(* Logix 5000 Routine export SpecLink_Routine; software revision 36.00 *)

TYPE DUT_NDSN_spLink :   // UDDT that holds the Cyclic and ACyclic data for the SpectraLink.
STRUCT
   b_r_LostComm : BOOL;
   b_r_PLC_CommReadOnly : BOOL;
   b_r_SystemReady : BOOL;   // Pattern Status Word 0 Bit 0
   b_r_Fault : BOOL;   // Pattern Status Word 0 Bit 1
   b_r_Alert : BOOL;   // Pattern Status Word 0 Bit 2
   b_r_Commissioned : BOOL;   // Pattern Status Word 0 Bit 3
   b_r_RecipeModified : BOOL;   // Pattern Status Word 0 Bit 5
   i_r_Recipe : INT;
   i_r_PalletizedCount : INT;
   i_r_PalletizedSkipCount : INT;
   di_r_App_Trig_ProductCount : DINT;
   di_r_FeedCount : DINT;
   di_r_DeliveryCount : DINT;
   st_r_AppStat : DUT_NDSN_spLink_Chan_Status[8];
   st_r_TrigStat : DUT_NDSN_spLink_Trig_Status[8];
   st_r_EncoStat : DUT_NDSN_spLink_Encoder_Status[8];
   i_r_ProductLength : DINT[8];
   i_r_ProdRate : INT;
   i_r_LineSpeed : INT[2];   // m/min units
   i_r_RunupOutput : INT[2];
   b_w_UnitEnable : BOOL;   // Pattern Control Word 0 Bit 0
   b_w_ClearAllAlarms : BOOL;   // Clear all System Faults and Alerts (Rising Edge).
   b_w_ResetAllCounters : BOOL;   // Reset all counters (rising edge).
   i_w_LoadRecipe : INT;
   i_w_PalletizedCount : INT;   // Write 0 to decrement; 1 to increment; 2 to reset; else does nothing.
   i_w_PalletizedSkipCount : INT;   // Write 0 to decrement; 1 to increment; 2 to reset; else does nothing.
   di_w_App_Trig_ProductCount : DINT;
   di_w_FeedCountReset : DINT;
   di_w_DeliveryCountReset : DINT;
   st_w_AppCtl : DUT_NDSN_spLink_Chan_CTL[8];
   st_rw_BeadAgg : DUT_NDSN_spLink_Bead[8];
   i_rw_RnUpPercentOutP1 : INT[2];
   i_rw_RnUpLineSpdP1 : INT[2];
   i_rw_RnUpPercentOutP2 : INT[2];
   i_rw_RnUpLineSpdP2 : INT[2];
   i_rw_RnUpLowLim : INT[2];
   i_rw_RnUpHighLim : INT[2];
   di_rw_EncoderRes : DINT[2];
   i_rw_TriggerMaskDist : DINT[8];
   i_rw_TriggerChCtl : INT[8];
   i_rw_EncoderChCtl : INT[2];
   i_rw_RandAdjStart : INT[8];
   i_rw_RandAdjEnd : INT[8];
   i_rw_VirtualTriggerSize : DINT[8];
   i_rw_ContStartSpeed : INT[8];
   i_rw_ContStopSpeed : INT[8];
   i_rw_ContKnifeCutDelay : DINT[8];
   i_rw_ContKnifeCutGap : DINT[8];
   di_rw_GTO : DINT[8];
   i_r_ErrorInfo : INT[4];
   i_r_SpecCtl : INT[4];
   i_r_CurrentFault : INT;
END_STRUCT
END_TYPE

TYPE DUT_NDSN_spLink_Bead :
STRUCT
   di_rw_NumOfBeads : DINT;
   di_rw_BeadDelay : DINT[8];   // 1/4 mm
   di_rw_BeadDuration : DINT[8];   // 1/4 mm
   di_rw_mode : DINT;   // 1/4 mm
   di_rw_MaxGunTime : DINT;   // microseconds
   di_rw_LineSpeedActivation : DINT;   // 100th m/min
   di_rw_LineSpeedDeactivation : DINT;   // 100th m/min
   di_rw_Interval : DINT;   // 1/4 mm
   di_rw_AdhesiveSavings : DINT;   // 30%-60%
   di_rw_EcoBeadPattern : DINT;   // 0-40, Illegal values: 0,1,11,20,21,30,31,38,39
END_STRUCT
END_TYPE

TYPE DUT_NDSN_spLink_Chan_CTL :
STRUCT
   b_w_Enable : BOOL;
   b_w_Purge : BOOL;
END_STRUCT
END_TYPE

TYPE DUT_NDSN_spLink_Chan_Status :
STRUCT
   b_r_Enabled : BOOL;
   b_r_Fault : BOOL;
   b_r_Alert : BOOL;
   b_r_Output_Active : BOOL;
   b_r_Installed : BOOL;
END_STRUCT
END_TYPE

TYPE DUT_NDSN_spLink_Encoder_Status :   // SpectraLink Encoder Channel Status
STRUCT
   b_r_Missing : BOOL;
   b_r_Phase_Missing : BOOL;
   b_r_Scaled : BOOL;
   b_r_Fault : BOOL;
   b_r_Alert : BOOL;
   b_r_Installed : BOOL;
END_STRUCT
END_TYPE

TYPE DUT_NDSN_spLink_HMI_Data :
STRUCT
   r_w_RunUp_1_P1_LineSpeed : REAL;
   r_w_RunUp_2_P1_LineSpeed : REAL;
   r_w_RunUp_1_P2_LineSpeed : REAL;
   r_w_RunUp_2_P2_LineSpeed : REAL;
   r_tempstorage : REAL[4];
   i_tempstorage : INT[4];
END_STRUCT
END_TYPE

TYPE DUT_NDSN_spLink_Rd_Wt :
STRUCT
   i_arr_ReadValue : INT[60];
   i_ReadADI : INT;
   b_ReadDone : BOOL;
   i_arr_WriteValue : INT[60];
   i_WriteADI : INT;
   i_WriteSizeBytes : INT;
   b_WriteEvent : BOOL;
   b_WriteDone : BOOL;
   b_FirstScan : BOOL;
   b_AllowWrites : BOOL;
   b_WriteErr : BOOL;
   b_ReadErr : BOOL;
END_STRUCT
END_TYPE

TYPE DUT_NDSN_spLink_Trig_Status :   // SpectraLink Trigger Channel Status
STRUCT
   b_r_Detected : BOOL;
   b_r_Fault : BOOL;
   b_r_Alert : BOOL;
   b_r_Active : BOOL;
   b_r_Installed : BOOL;
END_STRUCT
END_TYPE

TYPE DUT_spLink_ADI :
STRUCT
   i_ADI : INT;
   i_Size : INT;
END_STRUCT
END_TYPE

ADD_ON_INSTRUCTION AOI_spLink   (* revision 1.0 *)
// AOI to handle the I/O based data (Default Data) and Acyclic Data (low Priority) from the SpectraLink Pattern Controller.
VAR_IN_OUT
   IO_Input : INT[64]; {required}
   IO_Out : INT[64]; {required}
   spLink_HMI : DUT_NDSN_spLink; {required}
   IO_AcycRdWt : DUT_NDSN_spLink_Rd_Wt; {required}
   ReadMsg : MESSAGE; {required}
   WriteMsg : MESSAGE; {required}
   Read_Buffer : INT[100]; {required}
   Write_Buffer : INT[100]; {required}
END_VAR
VAR
   st_ADI_List : DUT_spLink_ADI[40]; {access None}
   tm_Command : FBD_TIMER; {access None}
   tm_Acyc : FBD_TIMER; {access None}
   b_AdhesiveOn : BOOL; {access None}
   b_AdhesiveOff : BOOL; {access None}
   b_Read : BOOL; {access None}
   i_ADI_Range : INT; {access None}
   i_ADI_Size : INT := 20; {access None}
   i_CompareIndex : INT; {access None}
   i_Index : INT; {access None}
   i_Index_Write : INT; {access None}
   i_rwADI_Count : INT := 12; {access None}
   i_rwDataSize : INT := 24; {access None}
   i_Size : INT; {access None}
   i_SizeofStruct : INT := 48; {access None}
   i_ValueIndex : INT; {access None}
   i : INT; {access None}
   i_temp_CPC : INT; {access None}
   arr_WriteIndex : DINT[40]; {access None}
   arr_WriteStartingAddress : DINT[40]; {access None}
   b_AcycWT_Rising : BOOL; {access None}
   arr_HMI : INT[600]; {access None}
   arr_HMI_Buffer : INT[600]; {access None}
   arr_HMI_Compare : INT[600]; {access None}
   b_AcycRD_Rising : BOOL; {access None}
   b_CommandRising : BOOL; {access None}
   tm_PalletizedCount_Reset : FBD_TIMER; {access None}
   b_ResetCurrentPalletizedCount : BOOL; {access None}
   b_ResetCurrentPalletizedSkipCount : BOOL; {access None}
   tm_PalletizedSkipCount_Reset : FBD_TIMER; {access None}
   i_temp_CPSC : INT; {access None}
   i_LoopCnt : INT; {access None}
   b_ResetSelectCount : BOOL; {access None}
   tm_ResetSelectCount : FBD_TIMER := (PRE := 5000); {access None}
   TRUE : BOOL := 1; {access None}
   FALSE : BOOL; {access None}
   tm_ResetFeedCount : FBD_TIMER; {access None}
   tm_ResetDeliveryCount : FBD_TIMER; {access None}
   i_WriteSizeTemp : INT; {access None}
   i_ReadADI_Temp : INT; {access None}
   tm_WriteEvent : FBD_TIMER; {access None}
   b_WriteEventONS : BOOL; {access None}
   i_WritePtr : DINT; {access None}
   Read_Watchdog : FBD_TIMER; {access None}
   Read_Time_Tic : FBD_TIMER; {access None}
   DINT_TEMP : DINT; {access None}
   DINT_Offset : INT; {access Read Only}
END_VAR

ROUTINE Logic   (* structured text *)
   //
   //		SpectraLink Add-On Instruction used to read/write Cyclic (high priority I/O)
   //		and Acyclic (low priority) data.
   //
   //
   //*******************************************************************************
   //	Initialize Code
   //*******************************************************************************
   
   IF IO_AcycRdWt.b_FirstScan THEN
   	i_ADI_Size:= 29;
   	i_rwADI_Count :=26;
   	i_SizeofStruct := 531;
   	i_rwDataSize := 522;
   	i_ADI_Range := 0;
   	i_ValueIndex :=0;
   	i_Index:=0;
   	IO_AcycRdWt.b_FirstScan := 0;		//Reset the FirstScan bit sent to the ADI from the main routine.
   	IO_AcycRdWt.b_AllowWrites := 0;		//Cycle through the full Read Data Set before allowing Writes to occur.  This populates the write compare buffers.
   
   	FOR i := 0 TO i_rwADI_Count DO
   		i_ADI_Range := i_ADI_Range + st_ADI_List[i].i_Size;
   		arr_WriteIndex[i] := i_ADI_Range;					//Index of all Read/Write ADI
   		arr_WriteStartingAddress[i + 1] := i_ADI_Range;		//All Read/Write ADI Starting Address
   	END_FOR;
   
   
   END_IF;
   
   
   
   
   //*******************************************************************************
   //  Start of Cyclic Data Code
   //
   //	The following code handles the I/O data for the High Priority DEFAULT ADIs.
   //*******************************************************************************
   
   // SpectraLink system Status
   spLink_HMI.b_r_SystemReady := IO_Input[0].0;
   spLink_HMI.b_r_Fault := IO_Input[0].1;
   spLink_HMI.b_r_Alert := IO_Input[0].2;
   spLink_HMI.b_r_Commissioned := IO_Input[0].3;
   spLink_HMI.b_r_PLC_CommReadOnly := IO_Input[0].4;
   spLink_HMI.b_r_RecipeModified := IO_Input[0].5;
   
   spLink_HMI.i_r_Recipe := IO_Input[4];
   spLink_HMI.i_r_PalletizedCount := IO_Input[5];
   spLink_HMI.i_r_PalletizedSkipCount := IO_Input[6];
   
   COP(IO_Input[7], spLink_HMI.di_r_App_Trig_ProductCount, 6);
   
   // Copy the Applicator Status Structure Bits from the IO_Inputs
   i_LoopCnt := 0;
   While (i_LoopCnt < 8) DO
   	spLink_HMI.st_r_AppStat[i_LoopCnt].b_r_Enabled := IO_Input[13+i_LoopCnt].0;
   	spLink_HMI.st_r_AppStat[i_LoopCnt].b_r_Fault := IO_Input[13+i_LoopCnt].1;
   	spLink_HMI.st_r_AppStat[i_LoopCnt].b_r_Alert := IO_Input[13+i_LoopCnt].2;
   	spLink_HMI.st_r_AppStat[i_LoopCnt].b_r_Output_Active := IO_Input[13+i_LoopCnt].3;
   	spLink_HMI.st_r_AppStat[i_LoopCnt].b_r_Installed := IO_Input[13+i_LoopCnt].4;
   	i_LoopCnt := i_LoopCnt+1;
   end_while;
   
   // Copy the Trigger Status Structure Bits from the IO_Inputs
   i_LoopCnt := 0;
   While (i_LoopCnt < 8) DO
   	spLink_HMI.st_r_TrigStat[i_LoopCnt].b_r_Detected := IO_Input[21+i_LoopCnt].0;
   	spLink_HMI.st_r_TrigStat[i_LoopCnt].b_r_Fault := IO_Input[21+i_LoopCnt].1;
   	spLink_HMI.st_r_TrigStat[i_LoopCnt].b_r_Alert := IO_Input[21+i_LoopCnt].2;
   	spLink_HMI.st_r_TrigStat[i_LoopCnt].b_r_Active := IO_Input[21+i_LoopCnt].3;
   	i_LoopCnt := i_LoopCnt+1;
   end_while;
   
   // Copy the Encoder Status Structure Bits from the IO_Inputs
   i_LoopCnt := 0;
   While (i_LoopCnt < 2) DO
   	spLink_HMI.st_r_EncoStat[i_LoopCnt].b_r_Missing := IO_Input[29+i_LoopCnt].0;
   	spLink_HMI.st_r_EncoStat[i_LoopCnt].b_r_Phase_Missing := IO_Input[29+i_LoopCnt].1;
   	spLink_HMI.st_r_EncoStat[i_LoopCnt].b_r_Scaled := IO_Input[29+i_LoopCnt].2;
   	spLink_HMI.st_r_EncoStat[i_LoopCnt].b_r_Fault := IO_Input[29+i_LoopCnt].3;
   	spLink_HMI.st_r_EncoStat[i_LoopCnt].b_r_Alert := IO_Input[29+i_LoopCnt].4;
   	i_LoopCnt := i_LoopCnt+1;
   end_while;
   
   
   //******************************************************************************************************************
   //Adjust the Product Length by a factor of 4
   //******************************************************************************************************************
   
   i_LoopCnt := 0;
   While (i_LoopCnt < 8) DO
   	DINT_Offset := i_LoopCnt*2;
   	COP(IO_Input[31+DINT_Offset], DINT_TEMP, 2);
   	spLink_HMI.i_r_ProductLength[i_LoopCnt] := (DINT_TEMP/4);
   	i_LoopCnt := i_LoopCnt+1;
   end_while;
   
   
   COP(IO_Input[47], spLink_HMI.i_r_ProdRate, 1);
   COP(IO_Input[48], spLink_HMI.i_r_LineSpeed[0], 2);
   COP(IO_Input[50], spLink_HMI.i_r_RunupOutput[0], 2);
   
   
   //******************************************************************************************************************
   //Cyclic WRITE Section
   //******************************************************************************************************************
   
   IO_Out[0].0 := spLink_HMI.b_w_UnitEnable;
   IO_Out[2].0 := spLink_HMI.b_w_ClearAllAlarms;
   IO_Out[2].1 := spLink_HMI.b_w_ResetAllCounters;
   
   IO_Out[4] := spLink_HMI.i_w_LoadRecipe;
   
   
   //********************************************************************************************************************************
   //Current Palatized Count & Current Palatized Skip Count     increment (1) or decrement (0);  else = other value     (ADI 16359 Write)
   //********************************************************************************************************************************
   //*********************************************************************
   //PLC logic will set the increment flag (1) or the decrement flag (0) which will generate a 1 second pulse to the spLink.  The
   //command must be set to a "else value" before another increment or decrement can occur.
   //*********************************************************************
   
   IF (spLink_HMI.i_w_PalletizedCount <> i_temp_CPC) AND NOT tm_PalletizedCount_Reset.EN AND NOT b_ResetCurrentPalletizedCount then
   	b_ResetCurrentPalletizedCount := 1;
   	i_temp_CPC := spLink_HMI.i_w_PalletizedCount;
   	tm_PalletizedCount_Reset.Reset := NOT b_ResetCurrentPalletizedCount;
   end_if;
   
   tm_PalletizedCount_Reset.PRE :=2000;
   tm_PalletizedCount_Reset.TimerEnable := b_ResetCurrentPalletizedCount;
   TONR(tm_PalletizedCount_Reset);
   
   If tm_PalletizedCount_Reset.DN then
   	b_ResetCurrentPalletizedCount := 0;
   end_if;
   
   
   IF (tm_PalletizedCount_Reset.EN AND NOT tm_PalletizedCount_Reset.DN AND (i_temp_CPC = 0)) then
   	IO_Out[5] := 0;
   elsif (tm_PalletizedCount_Reset.EN AND NOT tm_PalletizedCount_Reset.DN AND (i_temp_CPC = 1)) then
   	IO_Out[5] := 1;
   else
   	IO_Out[5] := 5;  // anything but a 1 or 0
   end_if;
   
   
   IF (spLink_HMI.i_w_PalletizedSkipCount <> i_temp_CPSC) AND NOT tm_PalletizedSkipCount_Reset.EN AND NOT b_ResetCurrentPalletizedSkipCount then
   	b_ResetCurrentPalletizedSkipCount := 1;
   	i_temp_CPSC := spLink_HMI.i_w_PalletizedSkipCount;
   	tm_PalletizedCount_Reset.Reset := NOT b_ResetCurrentPalletizedSkipCount;
   end_if;
   
   tm_PalletizedSkipCount_Reset.PRE :=2000;
   tm_PalletizedSkipCount_Reset.TimerEnable := b_ResetCurrentPalletizedSkipCount;
   TONR(tm_PalletizedSkipCount_Reset);
   
   IF (tm_PalletizedSkipCount_Reset.EN AND NOT tm_PalletizedSkipCount_Reset.DN AND (i_temp_CPSC = 0)) then
   	IO_Out[6] := 0;
   elsif (tm_PalletizedSkipCount_Reset.EN AND NOT tm_PalletizedSkipCount_Reset.DN AND (i_temp_CPSC = 1)) then
   	IO_Out[6] := 1;
   else
   	IO_Out[6] := 5;  // anything but a 1 or 0
   end_if;
   
   
   If tm_PalletizedSkipCount_Reset.DN then
   	b_ResetCurrentPalletizedSkipCount := 0;
   end_if;
   
   
   //********************************************************************************************************************************
   //Display Select Count, Feed Count and Delivery Count Reset     reset (1) or do nothing (0);        (ADI 16656 Write)
   //********************************************************************************************************************************
   //*********************************************************************
   //PLC logic will set the Reset (1) which will generate a 1 second pulse to the spLink.  The
   //command must be set to a "0" before another Reset can occur.
   //*********************************************************************
   
   
   	tm_ResetSelectCount.PRE := 1000;
   	tm_ResetSelectCount.TimerEnable := spLink_HMI.di_w_App_Trig_ProductCount.0;
   	tm_ResetSelectCount.Reset := NOT spLink_HMI.di_w_App_Trig_ProductCount.0;
   	TONR(tm_ResetSelectCount);
   
   	IF tm_ResetSelectCount.TT then
   		IO_Out[7] := 1;
   	else
   		IO_Out[7] := 0;
   	end_if;
   
   
   	tm_ResetFeedCount.PRE := 1000;
   	tm_ResetFeedCount.TimerEnable := spLink_HMI.di_w_FeedCountReset.0;
   	tm_ResetFeedCount.Reset := NOT spLink_HMI.di_w_FeedCountReset.0;
   	TONR(tm_ResetFeedCount);
   
   	IF tm_ResetFeedCount.TT then
   		IO_Out[9] := 1;
   	else
   		IO_Out[9] := 0;
   	end_if;
   
   
   	tm_ResetDeliveryCount.PRE := 1000;
   	tm_ResetDeliveryCount.TimerEnable := spLink_HMI.di_w_DeliveryCountReset.0;
   	tm_ResetDeliveryCount.Reset := NOT spLink_HMI.di_w_DeliveryCountReset.0;
   	TONR(tm_ResetDeliveryCount);
   
   	IF tm_ResetDeliveryCount.TT then
   		IO_Out[11] := 1;
   	else
   		IO_Out[11] := 0;
   	end_if;
   
   
   //********************************************************************************************************************************
   //Send the Applicator Channel Control Aggregate data to the PC.       (ADI 18675 Write)
   //********************************************************************************************************************************
   
   	i_LoopCnt := 0;
   While (i_LoopCnt < 8) DO
   	IO_Out[13+i_LoopCnt].0 := spLink_HMI.st_w_AppCtl[i_LoopCnt].b_w_Enable;
   	IO_Out[13+i_LoopCnt].1 := spLink_HMI.st_w_AppCtl[i_LoopCnt].b_w_Purge;
   	i_LoopCnt := i_LoopCnt+1;
   end_while;
   
   
   //*******************************************************************************************************************************
   //  Start of Acyclic Data Code
   //
   //	The following code handles the Explicit Messages for the Lower Priority ADIs.
   //*******************************************************************************
   
   tm_Acyc.PRE :=350;
   tm_Acyc.TimerEnable := NOT b_Read AND NOT IO_AcycRdWt.b_WriteEvent;
   TONR(tm_Acyc);
   b_Read :=tm_Acyc.DN;
   
   //Read Message Time Tic (25mSec between Reads)
   
   Read_Time_Tic.PRE := 25;
   Read_Time_Tic.TimerEnable := NOT Read_Time_Tic.DN;
   TONR(Read_Time_Tic);
   
   
   //Read Message Watchdog
   
   Read_Watchdog.PRE :=500;
   Read_Watchdog.TimerEnable := NOT Read_Watchdog.DN;
   TONR(Read_Watchdog);
   Read_Watchdog.Reset := 0;
   
   If Read_Watchdog.DN then
   	i_ReadADI_Temp  := 0;
   
   end_if;
   
   
   //******************************************************************
   //Sequentially read ALL ADIs and store into structure
   //b_read will initiate when tm_Acyc Expired,b_AcycRD_Tick will
   //trigger the funciton block when read is done,
   //b_AcycRD_Enable only last during Acyclic reading in process
   //When last ADI been read, it will stop reading until next cycle
   //*******************************************************************
   IO_AcycRdWt.i_ReadADI := st_ADI_List[i_Index].i_ADI;
   i_Size := st_ADI_List[i_Index].i_Size;
   
   
   If (IO_AcycRdWt.i_ReadADI <> i_ReadADI_Temp) AND Read_Time_Tic.DN then
   
   	ReadMsg.Instance := IO_AcycRdWt.i_ReadADI;
   	MSG(ReadMsg);
   	i_ReadADI_Temp := IO_AcycRdWt.i_ReadADI;
   
   end_if;
   
   IO_AcycRdWt.b_ReadDone := ReadMsg.DN;
   IO_AcycRdWt.b_ReadErr := ReadMsg.ER;
   
   IF IO_AcycRdWt.b_ReadDone AND NOT IO_AcycRdWt.b_WriteEvent AND b_AcycRD_Rising THEN
   
   	COP(Read_Buffer[0],arr_HMI[i_ValueIndex],i_Size);
   
   	//****************************************************
   	//After reading the current ADI, index to next one
   	//****************************************************
   	i_ValueIndex := i_ValueIndex + st_ADI_List[i_Index].i_Size;
       i_Index := i_Index + 1;
   
   	Read_Watchdog.Reset := 1;
   
   END_IF;
   
   b_AcycRD_Rising := NOT IO_AcycRdWt.b_ReadDone;
   
   
   //****************************************************
   //Copy all reading value into structure
   //****************************************************
   IF b_Read THEN
   	COP(arr_HMI[0],spLink_HMI.st_rw_BeadAgg[0],i_SizeofStruct);
   	COP(arr_HMI[0],arr_HMI_Buffer[0],i_rwDataSize);
   END_IF;
   
   IF ((i_Index = i_ADI_Size) AND b_Read) THEN
       i_Index := 0;
   	i_ValueIndex :=0;
   	IO_AcycRdWt.b_AllowWrites := 1;
   END_IF;
   
   //**********************************************************************************************
   //Copy all read/write ADI reading into arr_HMI_Buffer_Compare for further generating Write Event
   //***********************************************************************************************
   COP(spLink_HMI.st_rw_BeadAgg[0],arr_HMI_Compare[0],i_rwDataSize);
   
   //**************************************************************************************
   //Compare arr_HMI_Compare with arr_HMI_Buffer to generate write event
   //**************************************************************************************
   tm_WriteEvent.PRE :=350;
   tm_WriteEvent.TimerEnable :=IO_AcycRdWt.b_WriteEvent;
   TONR(tm_WriteEvent);
   
   
   b_WriteEventONS := 0;
   
   FOR i:=0 TO i_rwDataSize-1 BY 1 DO
   	IF (arr_HMI_Compare[i] <> arr_HMI_Buffer[i]) AND NOT IO_AcycRdWt.b_WriteEvent and IO_AcycRdWt.b_AllowWrites THEN
   
   		i_CompareIndex := i;
   		IO_AcycRdWt.b_WriteEvent := 1;
   		b_WriteEventONS := 1;
   		arr_HMI_Buffer[i] :=arr_HMI_Compare[i];
   
   		EXIT;
   	END_IF;
   END_FOR;
   
   IF b_WriteEventONS THEN
   	//***************************************************************
   	//When write event locate the write index inside arr_WriteIndex
   	//***************************************************************
       FOR i := 0 TO i_rwADI_Count DO
           IF i_CompareIndex < arr_WriteIndex[i] THEN
               i_Index_Write := i;
               EXIT;
           END_IF;
       END_FOR;
   
   	i_WriteSizeTemp := st_ADI_List[i_Index_Write].i_Size;
   	IO_AcycRdWt.i_WriteADI := st_ADI_List[i_Index_Write].i_ADI;
   
   	i_WritePtr := arr_WriteStartingAddress[i_Index_Write];
   	COP(arr_HMI_Compare[i_WritePtr],IO_AcycRdWt.i_arr_WriteValue[0],i_WriteSizeTemp);
   	COP(arr_HMI_Compare[i_WritePtr],arr_HMI[i_WritePtr],i_WriteSizeTemp);
   
   	IO_AcycRdWt.i_WriteSizeBytes := i_WriteSizeTemp*2;
   
   	COP(arr_HMI_Compare[i_WritePtr], Write_Buffer[0],i_WriteSizeTemp);
   	WriteMsg.Instance := IO_AcycRdWt.i_WriteADI;
   	WriteMsg.REQ_LEN := IO_AcycRdWt.i_WriteSizeBytes;
   	MSG(WriteMsg);
   
   END_IF;
   
   	IO_AcycRdWt.b_WriteDone := WriteMsg.DN;
   	IO_AcycRdWt.b_WriteErr := WriteMsg.ER;
   
   IF tm_WriteEvent.DN OR (IO_AcycRdWt.b_WriteDone AND b_AcycWT_Rising) THEN
   	IO_AcycRdWt.b_WriteEvent :=0;
   END_IF;
   b_AcycWT_Rising := NOT IO_AcycRdWt.b_WriteDone;
   
   
   
   
   //
   //   NOTES:  After MSG Write is working, go back and add ERR bits to the IO_AcycRdWt UDDT.
   //
   //
   
   
   
END_ROUTINE
END_ADD_ON_INSTRUCTION

VAR_GLOBAL   (* controller tags *)
   ADI_Temp_Constant : INT := 4;
   msg_AOI_spLink_Read : MESSAGE;
        MessageParameters(MessageType := CIP Generic, ConnectedFlag := 2, ConnectionPath := SpectraLink, ServiceCode := 16#000e, ObjectType := 16#00a2, TargetObject := 18692, AttributeNumber := 16#0005, DestinationTag := spLink_MSG_Read_Buffer)
   msg_AOI_spLink_Write : MESSAGE;
        MessageParameters(MessageType := CIP Generic, RequestedLength := 96, ConnectedFlag := 2, ConnectionPath := SpectraLink, ServiceCode := 16#0010, ObjectType := 16#00a2, TargetObject := 17274, AttributeNumber := 16#0005, LocalElement := spLink_MSG_Write_Buffer[0])
   msgRead_spLink : MESSAGE;
        MessageParameters(MessageType := CIP Generic, ConnectedFlag := 2, ConnectionPath := SpectraLink, ServiceCode := 16#000e, ObjectType := 16#00a2, TargetObject := 18100, AttributeNumber := 16#0005, DestinationTag := Test_Read_Array[0])
   msgWrite_spLink : MESSAGE;
        MessageParameters(MessageType := CIP Generic, RequestedLength := 2, ConnectedFlag := 2, ConnectionPath := SpectraLink, ServiceCode := 16#0010, ObjectType := 16#00a2, TargetObject := 18100, AttributeNumber := 16#0005, LocalElement := ADI_Temp_Constant)
   spLink_AcyRdWt : DUT_NDSN_spLink_Rd_Wt := (i_ReadADI := 18677, i_arr_WriteValue[0] := 1, i_arr_WriteValue[2] := 4, i_arr_WriteValue[18] := 400, i_arr_WriteValue[34] := 5, i_arr_WriteValue[36] := 10000, i_arr_WriteValue[38] := 500, i_arr_WriteValue[40] := 300, i_arr_WriteValue[42] := 400, i_arr_WriteValue[44] := 30, i_arr_WriteValue[46] := 2, i_WriteADI := 17274, i_WriteSizeBytes := 96, b_AllowWrites := 1);
   spLink_AOI : AOI_spLink;
   spLink_HMI : DUT_NDSN_spLink;
   spLink_HMI_Data : DUT_NDSN_spLink_HMI_Data := (r_w_RunUp_1_P2_LineSpeed := 100.0, r_w_RunUp_2_P2_LineSpeed := 100.0, r_tempstorage[2] := 100.0, r_tempstorage[3] := 100.0, i_tempstorage[2] := 10000, i_tempstorage[3] := 10000);
   spLink_MSG_Read_Buffer : INT[100] := ([0] := 3, [1] := 3, [2] := 3, [3] := 3, [4] := 1, [5] := 1, [6] := 1, [7] := 1, [18] := 400, [34] := 4, [36] := 10000, [38] := 950, [40] := 450, [42] := 120, [44] := 30, [46] := 7);
   spLink_MSG_Write_Buffer : INT[100] := ([0] := 1, [2] := 4, [18] := 400, [34] := 5, [36] := 10000, [38] := 500, [40] := 300, [42] := 400, [44] := 30, [46] := 2);
   Test_Read_Array : INT[4];
   Test_Read_Data : INT := 4;
END_VAR

PROGRAM MainProgram
VAR
   i_splink_1_Comm : DINT := 16384;
   msgRead_ONS : BOOL;
   msgWrite_ONS : BOOL;
   Read_Temp : INT := 4;
   splink_CommLost_cnt : DINT;
   splink_LostComm_ONS : BOOL;
   Start_ReadMSG : BOOL;
   Start_WriteMSG : BOOL;
   Test_Read_Att : INT := 18100;
   Test_Write_Att : INT := 18100;
   Test_Write_Data : INT := 4;
   tm_spLink_CommStarting : TIMER := (PRE := 5000);
END_VAR

ROUTINE SpecLink_Routine   (* ladder *)
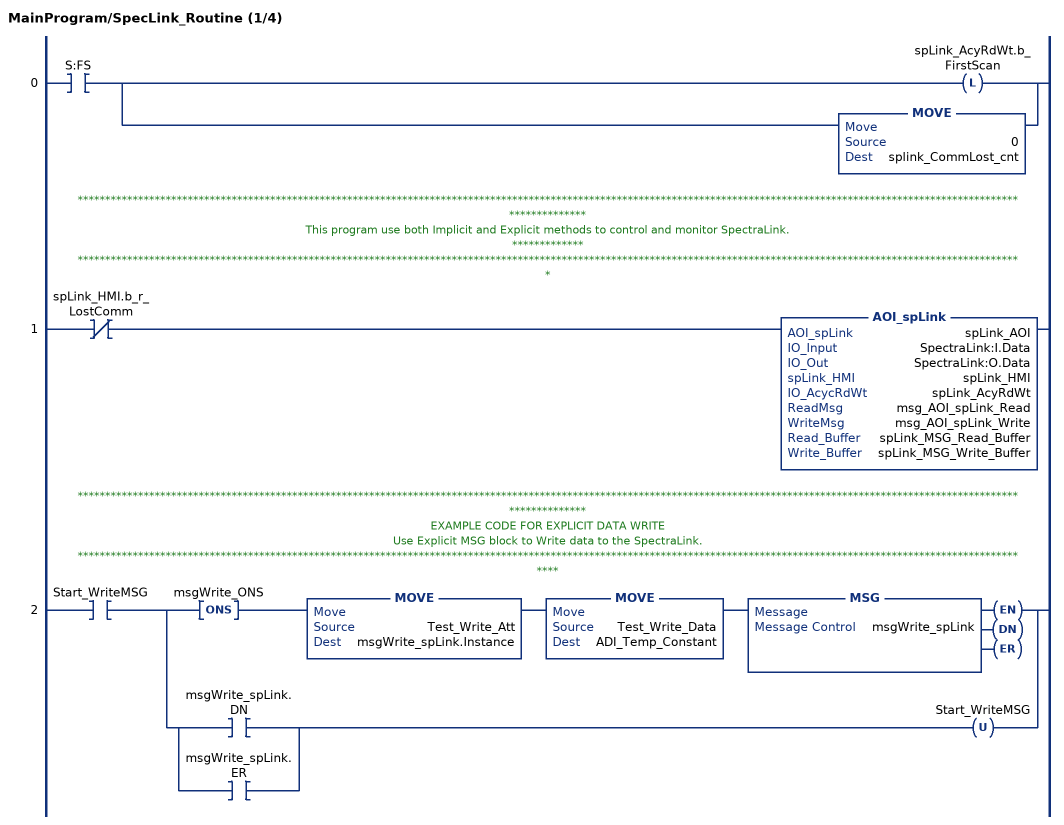
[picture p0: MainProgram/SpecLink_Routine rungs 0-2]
   0: XIC(S:FS)[OTL(spLink_AcyRdWt.b_FirstScan) ,MOVE(0,splink_CommLost_cnt) ];
   // *****************************************************************************************************************************************************************************************
   // This program use both Implicit and Explicit methods to control and monitor SpectraLink.
   // *************
   // ****************************************************************************************************************************************************************************
   1: XIO(spLink_HMI.b_r_LostComm)AOI_spLink(spLink_AOI,SpectraLink:I.Data,SpectraLink:O.Data,spLink_HMI,spLink_AcyRdWt,msg_AOI_spLink_Read,msg_AOI_spLink_Write,spLink_MSG_Read_Buffer,spLink_MSG_Write_Buffer);
   // *****************************************************************************************************************************************************************************************
   // EXAMPLE CODE FOR EXPLICIT DATA WRITE
   // Use Explicit MSG block to Write data to the SpectraLink.
   // *******************************************************************************************************************************************************************************
   2: XIC(Start_WriteMSG)[ONS(msgWrite_ONS) MOVE(Test_Write_Att,msgWrite_spLink.Instance) MOVE(Test_Write_Data,ADI_Temp_Constant) MSG(msgWrite_spLink) ,[XIC(msgWrite_spLink.DN) ,XIC(msgWrite_spLink.ER) ] OTU(Start_WriteMSG) ];
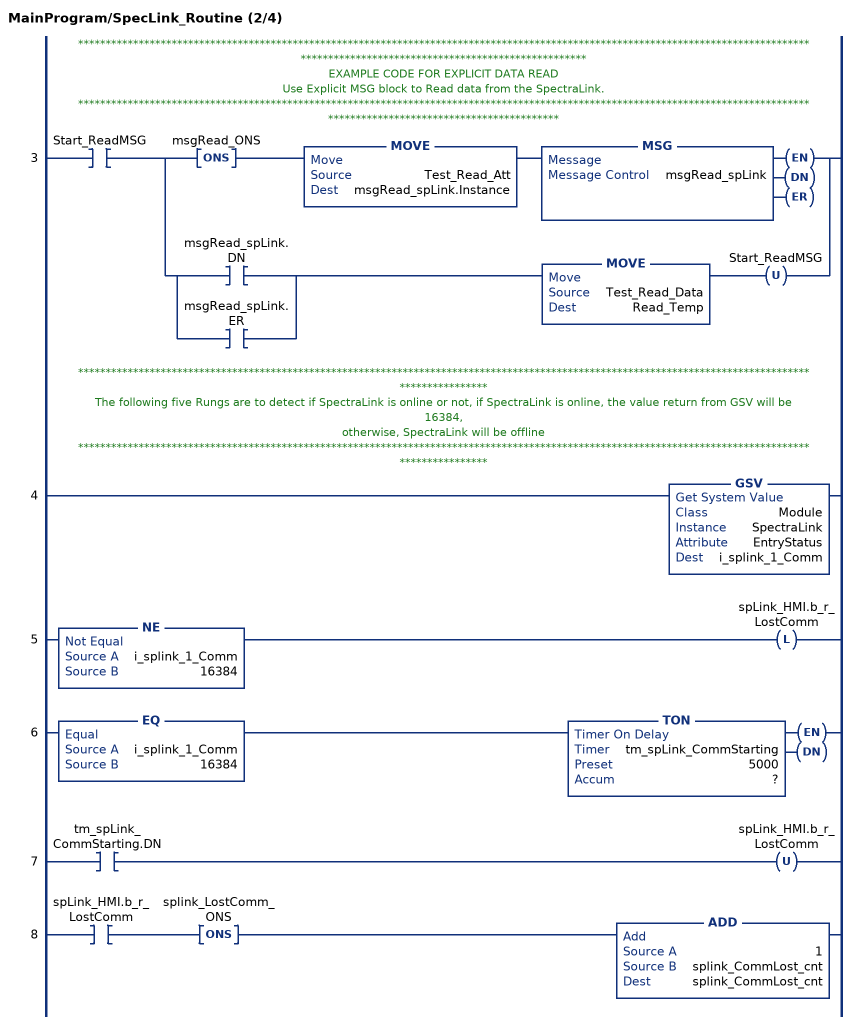
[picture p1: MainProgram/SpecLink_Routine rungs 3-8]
   // *****************************************************************************************************************************************************************************************
   // EXAMPLE CODE FOR EXPLICIT DATA READ
   // Use Explicit MSG block to Read data from the SpectraLink.
   // *******************************************************************************************************************************************************************************
   3: XIC(Start_ReadMSG)[ONS(msgRead_ONS) MOVE(Test_Read_Att,msgRead_spLink.Instance) MSG(msgRead_spLink) ,[XIC(msgRead_spLink.DN) ,XIC(msgRead_spLink.ER) ] MOVE(Test_Read_Data,Read_Temp) OTU(Start_ReadMSG) ];
   // *****************************************************************************************************************************************************
   // The following five Rungs are to detect if SpectraLink is online or not, if SpectraLink is online, the value return from GSV will be 16384,
   // otherwise, SpectraLink will be offline
   // *****************************************************************************************************************************************************
   4: GSV(Module,SpectraLink,EntryStatus,i_splink_1_Comm);
   5: NE(i_splink_1_Comm,16384)OTL(spLink_HMI.b_r_LostComm);
   6: EQ(i_splink_1_Comm,16384)TON(tm_spLink_CommStarting,?,?);
   7: XIC(tm_spLink_CommStarting.DN)OTU(spLink_HMI.b_r_LostComm);
   8: XIC(spLink_HMI.b_r_LostComm)ONS(splink_LostComm_ONS)ADD(1,splink_CommLost_cnt,splink_CommLost_cnt);
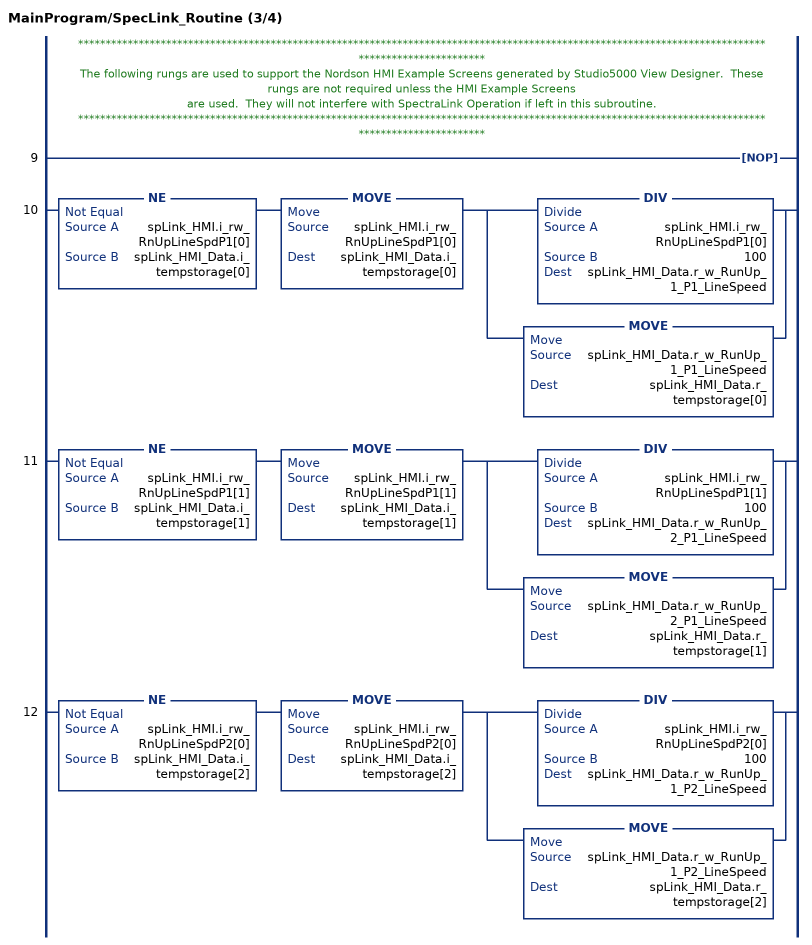
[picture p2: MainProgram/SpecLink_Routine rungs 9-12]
   // ****************************************************************************************************************************************************
   // The following rungs are used to support the Nordson HMI Example Screens generated by Studio5000 View Designer.  These rungs are not required unless the HMI Example Screens
   // are used.  They will not interfere with SpectraLink Operation if left in this subroutine.
   // ****************************************************************************************************************************************************
   9: NOP();
   10: NE(spLink_HMI.i_rw_RnUpLineSpdP1[0],spLink_HMI_Data.i_tempstorage[0])MOVE(spLink_HMI.i_rw_RnUpLineSpdP1[0],spLink_HMI_Data.i_tempstorage[0])[DIV(spLink_HMI.i_rw_RnUpLineSpdP1[0],100,spLink_HMI_Data.r_w_RunUp_1_P1_LineSpeed) ,MOVE(spLink_HMI_Data.r_w_RunUp_1_P1_LineSpeed,spLink_HMI_Data.r_tempstorage[0]) ];
   11: NE(spLink_HMI.i_rw_RnUpLineSpdP1[1],spLink_HMI_Data.i_tempstorage[1])MOVE(spLink_HMI.i_rw_RnUpLineSpdP1[1],spLink_HMI_Data.i_tempstorage[1])[DIV(spLink_HMI.i_rw_RnUpLineSpdP1[1],100,spLink_HMI_Data.r_w_RunUp_2_P1_LineSpeed) ,MOVE(spLink_HMI_Data.r_w_RunUp_2_P1_LineSpeed,spLink_HMI_Data.r_tempstorage[1]) ];
   12: NE(spLink_HMI.i_rw_RnUpLineSpdP2[0],spLink_HMI_Data.i_tempstorage[2])MOVE(spLink_HMI.i_rw_RnUpLineSpdP2[0],spLink_HMI_Data.i_tempstorage[2])[DIV(spLink_HMI.i_rw_RnUpLineSpdP2[0],100,spLink_HMI_Data.r_w_RunUp_1_P2_LineSpeed) ,MOVE(spLink_HMI_Data.r_w_RunUp_1_P2_LineSpeed,spLink_HMI_Data.r_tempstorage[2]) ];
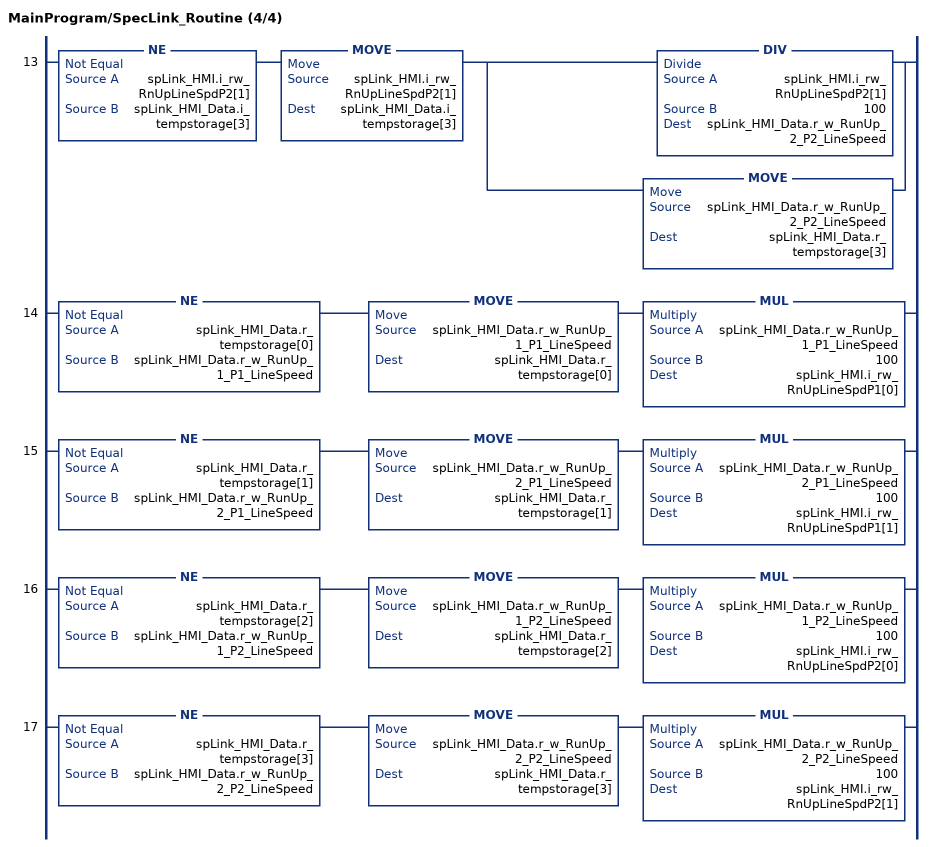
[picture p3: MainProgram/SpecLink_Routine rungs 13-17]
   13: NE(spLink_HMI.i_rw_RnUpLineSpdP2[1],spLink_HMI_Data.i_tempstorage[3])MOVE(spLink_HMI.i_rw_RnUpLineSpdP2[1],spLink_HMI_Data.i_tempstorage[3])[DIV(spLink_HMI.i_rw_RnUpLineSpdP2[1],100,spLink_HMI_Data.r_w_RunUp_2_P2_LineSpeed) ,MOVE(spLink_HMI_Data.r_w_RunUp_2_P2_LineSpeed,spLink_HMI_Data.r_tempstorage[3]) ];
   14: NE(spLink_HMI_Data.r_tempstorage[0],spLink_HMI_Data.r_w_RunUp_1_P1_LineSpeed)MOVE(spLink_HMI_Data.r_w_RunUp_1_P1_LineSpeed,spLink_HMI_Data.r_tempstorage[0])MUL(spLink_HMI_Data.r_w_RunUp_1_P1_LineSpeed,100,spLink_HMI.i_rw_RnUpLineSpdP1[0]);
   15: NE(spLink_HMI_Data.r_tempstorage[1],spLink_HMI_Data.r_w_RunUp_2_P1_LineSpeed)MOVE(spLink_HMI_Data.r_w_RunUp_2_P1_LineSpeed,spLink_HMI_Data.r_tempstorage[1])MUL(spLink_HMI_Data.r_w_RunUp_2_P1_LineSpeed,100,spLink_HMI.i_rw_RnUpLineSpdP1[1]);
   16: NE(spLink_HMI_Data.r_tempstorage[2],spLink_HMI_Data.r_w_RunUp_1_P2_LineSpeed)MOVE(spLink_HMI_Data.r_w_RunUp_1_P2_LineSpeed,spLink_HMI_Data.r_tempstorage[2])MUL(spLink_HMI_Data.r_w_RunUp_1_P2_LineSpeed,100,spLink_HMI.i_rw_RnUpLineSpdP2[0]);
   17: NE(spLink_HMI_Data.r_tempstorage[3],spLink_HMI_Data.r_w_RunUp_2_P2_LineSpeed)MOVE(spLink_HMI_Data.r_w_RunUp_2_P2_LineSpeed,spLink_HMI_Data.r_tempstorage[3])MUL(spLink_HMI_Data.r_w_RunUp_2_P2_LineSpeed,100,spLink_HMI.i_rw_RnUpLineSpdP2[1]);
END_ROUTINE
END_PROGRAM
